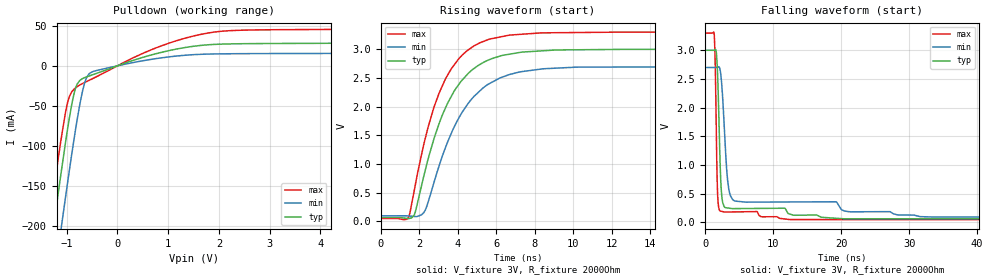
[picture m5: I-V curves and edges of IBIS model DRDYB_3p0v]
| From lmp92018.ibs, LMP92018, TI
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|   Model
[Model]   DRDYB_3p0v
Model_type   Open_drain
Polarity   Non-Inverting
Vmeas = 1.5
Vref = 3
Cref = 1pF
Rref = 2000
|   typ   min   max
C_comp   0.6389pF   0.6288pF   0.7669pF
[Voltage Range]   3   2.7   3.3
[Temperature Range]   27   125   -40
[Pullup Reference]   3   2.7   3.3
[Pulldown Reference]   0   0   0
[Power Clamp Reference]   3   2.7   3.3
[GND Clamp Reference]   0   0   0
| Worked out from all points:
|   slope of the pulldown table from 0 to 0.45 V, typ, clamps not added: 47 ohm
|   falling waveform, V_fixture 3V, R_fixture 2000Ohm: 20-80 % time 451ps typ, 866ps min, 278ps max; typ from 3 V to 0.064 V
|   rising waveform, V_fixture 3V, R_fixture 2000Ohm: 20-80 % time 1.97ns typ, 2.14ns min, 1.82ns max; typ from 0.064 V to 3 V
[Pulldown]
|   Voltage   I(typ)   I(min)   I(max)
-3V       -1.049A    -1.117A    -1.006A
-1.353V   -245.9mA   -317.1mA   -201.2mA
-1.335V   -237.4mA   -308.6mA   -192.8mA
-1.173V   -162.2mA   -232.8mA   -118.7mA
-1.119V   -137.8mA   -207.9mA   -95.37mA
-975mV    -76.12mA   -143mA     -44.25mA
-831mV    -29.14mA   -81.93mA   -27.85mA
-651mV    -14.91mA   -22.46mA   -21.04mA
-489mV    -11.18mA   -7.299mA   -16.03mA
771mV     15.31mA    9.097mA    22.67mA
1.851V    26.56mA    14.77mA    41.67mA
5.991V    28.79mA    15.93mA    46.2mA
[Ramp]
R_load = 2000
|   typ   min   max
dV/dt_r   1.76163/1.97187e-09   1.56323/2.14275e-09   1.951/1.81991e-09
dV/dt_f   1.76163/4.51089e-10   1.56323/8.66497e-10   1.951/2.77542e-10
[Falling Waveform]
V_fixture = 3V
V_fixture_min = 2.7V
V_fixture_max = 3.3V
R_fixture = 2000Ohm
C_fixture = 0F
|   Time   V(typ)   V(min)   V(max)
0s        3V         2.7V       3.3V
1.349ns   3.003V     2.7V       3.258V
1.504ns   3.014V     2.7V       2.624V
1.767ns   2.746V     2.705V     739.9mV
2.093ns   1.5V       2.701V     217.1mV
2.51ns    394.7mV    2.292V     190.5mV
3.177ns   254.3mV    906.5mV    181.8mV
3.738ns   245.2mV    459.9mV    182.8mV
12.47ns   145.9mV    357.2mV    50.58mV
300ns     63.95mV    94.61mV    48.33mV
[Rising Waveform]
V_fixture = 3V
V_fixture_min = 2.7V
V_fixture_max = 3.3V
R_fixture = 2000Ohm
C_fixture = 0F
|   Time   V(typ)   V(min)   V(max)
0s        63.95mV    94.61mV    48.33mV
1.434ns   44.87mV    91.61mV    59.91mV
1.788ns   156.2mV    82.1mV     623.8mV
2.236ns   788.5mV    149.7mV    1.343V
2.715ns   1.381V     619.6mV    1.935V
3.344ns   1.961V     1.269V     2.468V
4.033ns   2.375V     1.787V     2.825V
5.581ns   2.808V     2.388V     3.167V
8.306ns   2.969V     2.652V     3.283V
300ns     3V         2.7V       3.3V
